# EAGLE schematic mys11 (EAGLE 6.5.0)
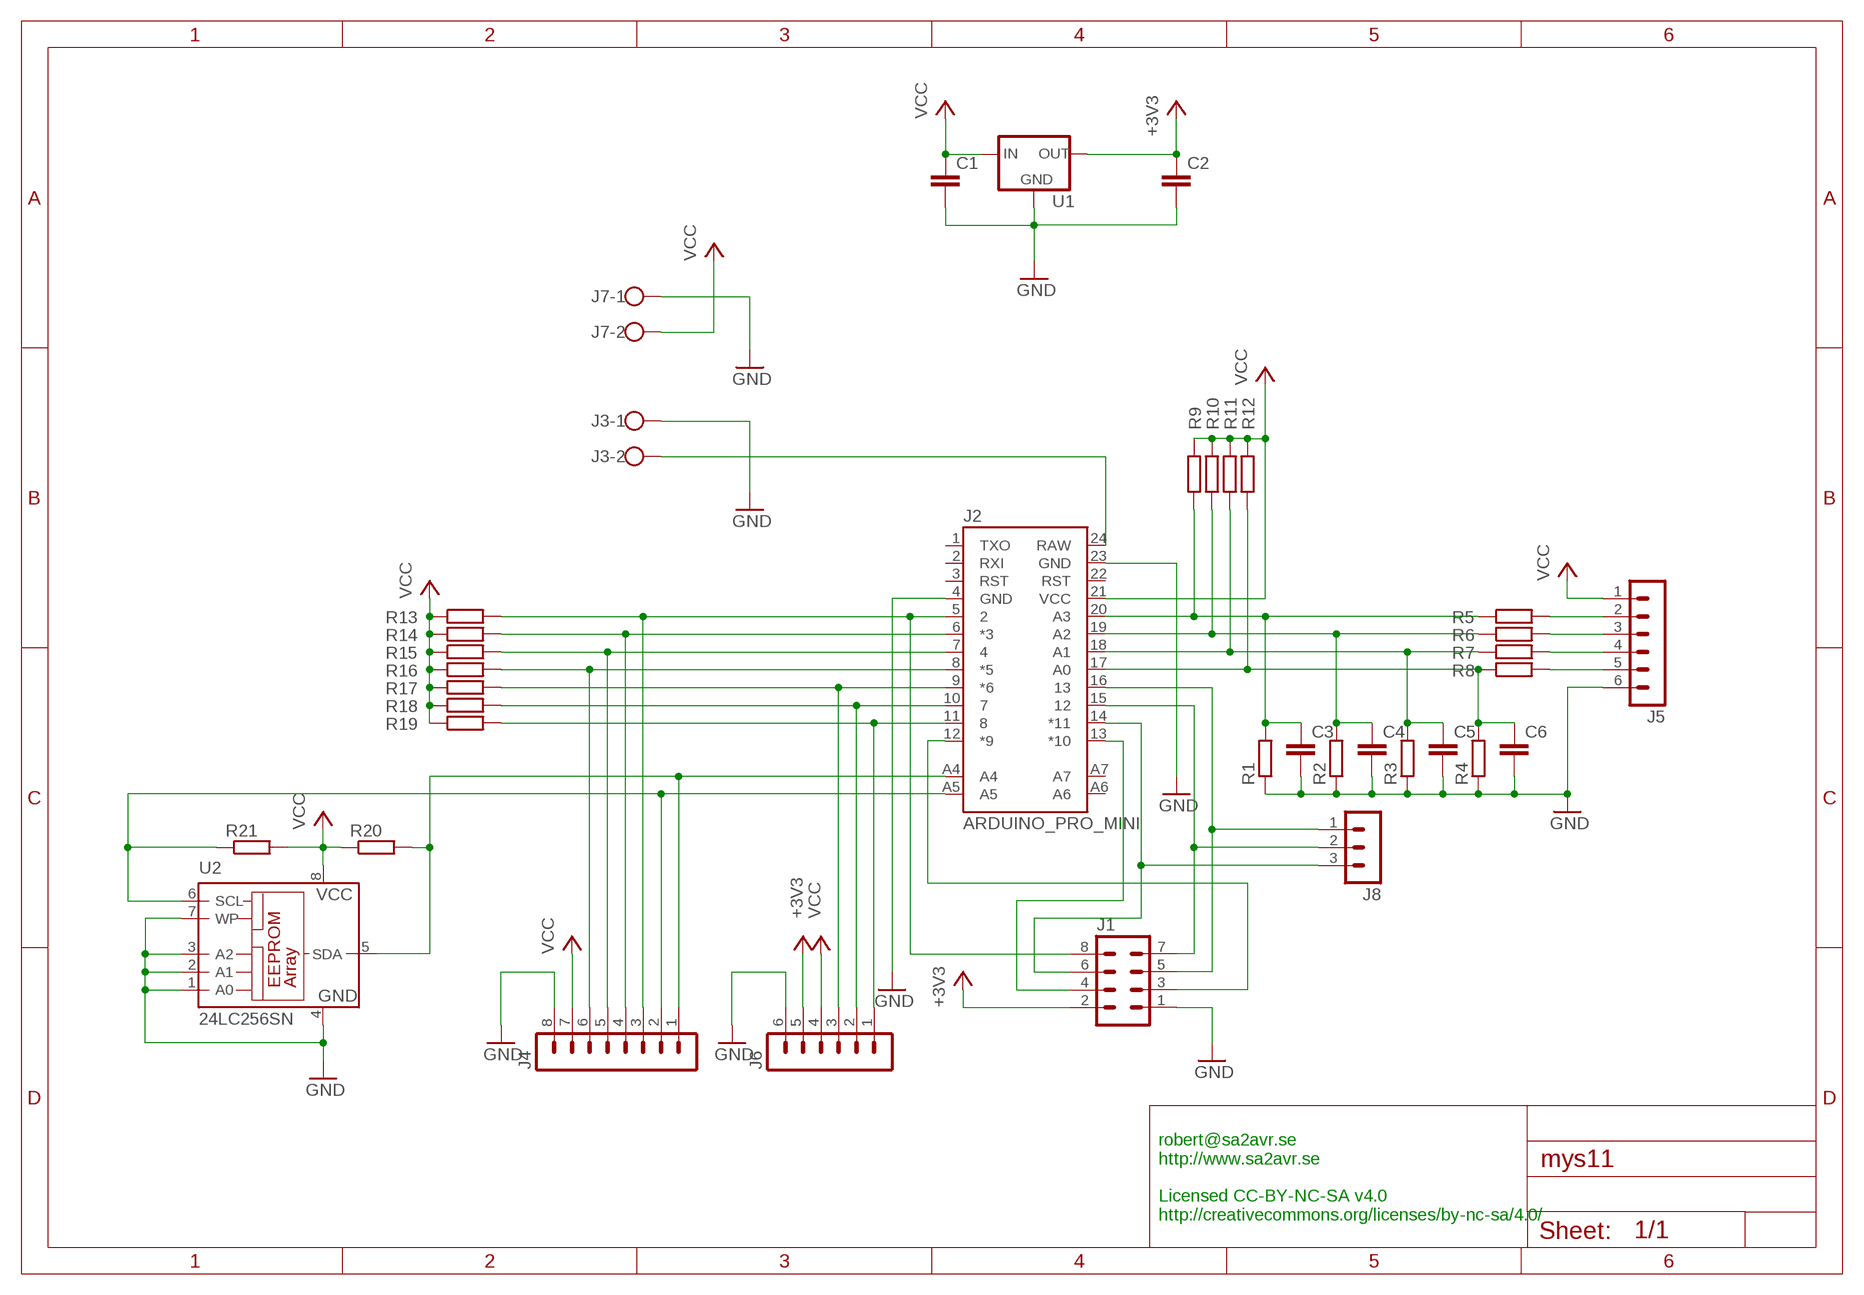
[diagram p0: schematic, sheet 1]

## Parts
C1  C-EUC0805  [C0805]
C2  C-EUC0805  [C0805]
C3  C-EUC0805  [C0805]
C4  C-EUC0805  [C0805]
C5  C-EUC0805  [C0805]
C6  C-EUC0805  [C0805]
J1  MA04-2  [MA04-2]
J2  ARDUINO_PRO_MINI  [ARDUINO_PRO_MINI]
J3  W237-102  [W237-102]
J4  MA08-1  [MA08-1]
J5  MA06-1  [MA06-1]
J6  MA06-1  [MA06-1]
J7  W237-102  [W237-102]
J8  MA03-1  [MA03-1]
R1  R-EU_R0805  [R0805]
R2  R-EU_R0805  [R0805]
R3  R-EU_R0805  [R0805]
R4  R-EU_R0805  [R0805]
R5  R-EU_R0805  [R0805]
R6  R-EU_R0805  [R0805]
R7  R-EU_R0805  [R0805]
R8  R-EU_R0805  [R0805]
R9  R-EU_R0805  [R0805]
R10  R-EU_R0805  [R0805]
R11  R-EU_R0805  [R0805]
R12  R-EU_R0805  [R0805]
R13  R-EU_R0805  [R0805]
R14  R-EU_R0805  [R0805]
R15  R-EU_R0805  [R0805]
R16  R-EU_R0805  [R0805]
R17  R-EU_R0805  [R0805]
R18  R-EU_R0805  [R0805]
R19  R-EU_R0805  [R0805]
R20  R-EU_R0805  [R0805]
R21  R-EU_R0805  [R0805]
U1  XC63FPM  [SOT23]
U2  24LC256SN  [SO-08]

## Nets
+3V3: C2.1 J1.2 J6.5 U1.2(OUT)
GND: C1.2 C2.2 C3.2 C4.2 C5.2 C6.2 J1.1 J2.4(GND) J2.23(GND) J3.1 J4.8 J5.6 J6.6 J7.1 R1.1 R2.1 R3.1 R4.1 U1.1(GND) U2.1(A0) U2.2(A1) U2.3(A2) U2.4(GND) U2.7(WP)
N$1: J1.8 J2.5 J4.3 R13.2
N$2: J2.6(*3) J4.4 R14.2
N$3: J2.7 J4.5 R15.2
N$4: J2.8(*5) J4.6 R16.2
N$5: J2.9(*6) J6.3 R17.2
N$6: J2.10 J6.2 R18.2
N$7: J2.11 J6.1 R19.2
N$8: C3.1 J2.20(A3) R1.2 R5.1 R9.1
N$9: C4.1 J2.19(A2) R2.2 R6.1 R10.1
N$10: C5.1 J2.18(A1) R3.2 R7.1 R11.1
N$11: C6.1 J2.17(A0) R4.2 R8.1 R12.1
N$12: J5.2 R5.2
N$13: J5.3 R6.2
N$14: J5.4 R7.2
N$15: J5.5 R8.2
N$16: J1.3 J2.12(*9)
N$17: J1.4 J2.13(*10)
N$18: J1.6 J2.14(*11) J8.3
N$19: J1.7 J2.15 J8.2
N$20: J1.5 J2.16 J8.1
N$21: J2.24(RAW) J3.2
N$22: J2.A4 J4.1 R20.2 U2.5(SDA)
N$23: J2.A5 J4.2 R21.1 U2.6(SCL)
VCC: C1.1 J2.21(VCC) J4.7 J5.1 J6.4 J7.2 R9.2 R10.2 R11.2 R12.2 R13.1 R14.1 R15.1 R16.1 R17.1 R18.1 R19.1 R20.1 R21.2 U1.3(IN) U2.8(VCC)
Unconnected: J2.1(TXO) J2.2(RXI) J2.3(RST) J2.22(RST) J2.A6 J2.A7

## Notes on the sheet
- robert@sa2avr.se
  http://www.sa2avr.se
  
  Licensed CC-BY-NC-SA v4.0
  http://creativecommons.org/licenses/by-nc-sa/4.0/

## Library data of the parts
C1-C6 = resistor:C-EU: CAPACITOR, European symbol
J1 = con-lstb:MA04-2: PIN HEADER; OC_FARNELL: unknown; OC_NEWARK: unknown
J2 = SparkFun-Boards:ARDUINO_PRO_MINI
J3 J7 = con-wago-500:W237-102: WAGO SCREW CLAMP; MPN: 237-102; OC_FARNELL: unknown; OC_NEWARK: 70K9898
J4 = con-lstb:MA08-1: PIN HEADER; OC_FARNELL: unknown; OC_NEWARK: unknown
J5 J6 = con-lstb:MA06-1: PIN HEADER; OC_FARNELL: unknown; OC_NEWARK: unknown
J8 = con-lstb:MA03-1: PIN HEADER; OC_FARNELL: unknown; OC_NEWARK: unknown
R1-R21 = resistor:R-EU_: RESISTOR, European symbol
U1 = v-reg:XC63FP: Positiv Voltage Regulators www.torex.co.jp/english/product/pro02/pdf/0201_xc62fp.pdf
U2 = microchip:24*: Serial EEPROM I2C; MF: MICROCHIP; MPN: 24LC256-I/SN; OC_FARNELL: 9757996; OC_NEWARK: 27C9144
